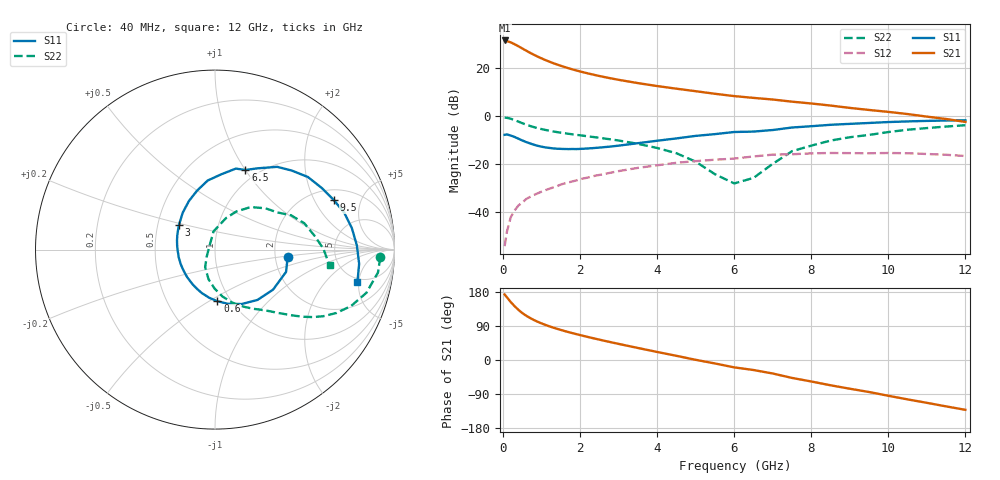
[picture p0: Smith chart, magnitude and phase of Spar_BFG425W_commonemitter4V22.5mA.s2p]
! Filename: 422bfg425.001
! BFG425W Field C1
! V1=8.377E-001V,V2=4.000E+000V, I1=2.768E-004A, I2=2.248E-002A
# GHz  S  MA  R 50
!  S11  S21  S12  S22
!Freq(GHz)  Mag  Ang  Mag  Ang  Mag  Ang  Mag  Ang
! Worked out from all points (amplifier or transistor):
!   44 points, 40 MHz to 12 GHz, reference 50 ohm
!   highest |S21| = 31.3 dB at 40 MHz (marker M1)
!   |S21| within 3 dB of that: start of sweep to 464 MHz
!   unconditionally stable (mu >= 1): start of sweep to 46.87 MHz; 1.271 GHz to end of sweep
!   at 700 MHz: K = 0.77, MSG = 29.9 dB, |S12| = -33.6 dB
!   at 2.4 GHz: K = 1.14, MAG = 18.6 dB, |S12| = -24.7 dB
!   at 12 GHz: K = 1.34, MAG = 3.6 dB, |S12| = -16.6 dB
!   S11 on the Smith chart (normalised r, x): 40 MHz: 2.35, -0.23; 600 MHz: 0.87, -0.54; 3 GHz: 0.64, +0.19; 6.5 GHz: 0.87, +1.00; 9.5 GHz: 2.54, +2.89; 12 GHz: 4.47, -4.80
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0.04  0.407 -5.7  36.83 173.0  0.002 52.5  0.922 -2.6
0.1  0.415 -17.4  35.75 165.4  0.004 76.3  0.917 -8.0
0.2  0.393 -34.5  33.62 152.8  0.008 73.1  0.877 -15.9
0.3  0.367 -49.8  30.78 141.9  0.011 70.0  0.821 -22.5
0.4  0.338 -63.7  27.87 132.3  0.014 67.5  0.763 -27.6
0.5  0.311 -76.4  25.12 123.8  0.016 64.8  0.709 -31.5
0.6  0.288 -87.4  22.62 116.8  0.019 63.5  0.662 -34.6
0.7  0.27 -97.0  20.47 110.9  0.021 62.1  0.622 -37.0
0.8  0.254 -106.2  18.61 105.5  0.023 61.4  0.588 -39.0
0.9  0.241 -114.4  17.02 100.8  0.025 60.8  0.56 -40.8
1  0.231 -122.0  15.63 96.5  0.027 60.1  0.535 -42.4
1.2  0.218 -135.6  13.4 88.9  0.031 58.9  0.496 -45.3
1.6  0.207 -158.7  10.35 76.4  0.04 56.3  0.439 -50.6
2.2  0.212 174.0  7.648 60.8  0.053 50.9  0.379 -59.2
3  0.243 145.7  5.625 42.5  0.072 41.7  0.31 -72.0
4.5  0.343 107.0  3.682 11.0  0.107 20.5  0.169 -102.3
5.5  0.421 85.2  2.888 -9.2  0.124 5.0  0.062 -138.7
6.5  0.475 69.1  2.374 -26.4  0.145 -7.2  0.052 116.8
8.5  0.657 38.0  1.646 -66.7  0.171 -44.2  0.309 50.1
9.5  0.717 22.7  1.334 -84.5  0.169 -61.0  0.405 30.7
10.5  0.772 8.9  1.097 -104.0  0.169 -79.7  0.519 16.4
12  0.814 -12.9  0.754 -131.5  0.148 -109.8  0.644 -7.9
